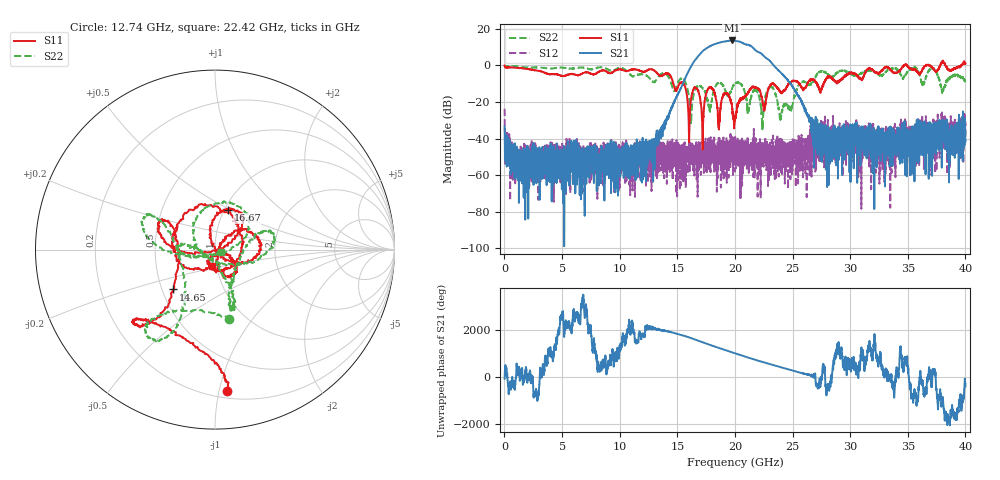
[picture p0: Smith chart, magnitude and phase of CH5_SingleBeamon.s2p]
!Keysight Technologies,N5245B,MY57181321,A.14.80.03
!Date: Thursday, March 28, 2024 19:43:59
!Correction: S11(C  2-Port  )
!S21(C  2-Port  )
!S12(C  2-Port  )
!S22(C  2-Port  )
!S2P File: Measurements: S11, S21, S12, S22:
# Hz S  RI  R 50
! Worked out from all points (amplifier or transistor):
!   4000 points, 10 MHz to 40 GHz, reference 50 ohm
!   highest |S21| = 13.7 dB at 19.73 GHz (marker M1)
!   |S21| within 3 dB of that: 17.88 GHz to 21.39 GHz (3.51 GHz wide, 17.9 % of centre)
!   unconditionally stable (mu >= 1): 15.4 MHz to 34.65 GHz; 34.96 GHz to 36.55 GHz; 38.27 GHz to 39.61 GHz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
!   at 6.67 GHz: K = 26125.73, MAG = -37.4 dB, |S12| = -65.4 dB
!   at 20.01 GHz: K = 76.01, MAG = 14.0 dB, |S12| = -58.1 dB
!   at 40 GHz: K = -267.43, MSG = -2.7 dB, |S12| = -30.6 dB
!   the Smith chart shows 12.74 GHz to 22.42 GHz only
!   S11 on the Smith chart (normalised r, x): 12.74 GHz: 0.25, -1.06; 14.65 GHz: 0.57, -0.28; 16.67 GHz: 1.04, +0.49; 22.42 GHz: 0.95, -0.17
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1e7  0.9943 -0.0372  0.00504 -0.0208  -0.055 0.0347  -0.9791 0.0426
6.68e9  0.2945 0.5044  -0.00285 -0.00276  -0.00171 -0.00146  0.8145 0.3385
1.274e10  0.0662 -0.7879  0.00294 -0.00392  -0.00284 0.000729  0.0805 -0.3877
1.334e10  -0.0625 -0.571  -0.00795 -0.0119  -0.000748 0.00354  -0.3036 -0.3661
1.465e10  -0.2313 -0.2218  -0.0057 0.0864  0.00161 -0.00291  -0.1835 -0.1164
1.611e10  0.0674 0.0272  -0.4226 -0.7262  0.00366 -0.00125  -0.0462 -0.0377
1.667e10  0.0734 0.2219  -1.217 1.015  -0.00259 0.00216  0.1898 0.1756
1.711e10  -0.0185 0.0458  1.125 2.017  -0.000644 -0.00199  -0.00339 0.2543
1.755e10  0.1736 -0.0702  2.863 -0.837  0.000278 0.00117  -0.119 0.0703
1.807e10  0.2062 0.0929  -1.03 -3.501  0.000312 -0.00505  0.1388 -0.0831
1.859e10  0.0193 0.00379  -4.067 0.9829  0.000737 -0.0101  0.3317 0.0573
1.914e10  0.0942 -0.1418  0.9517 4.452  -0.00117 -0.00257  0.208 0.062
1.973e10  0.076 -0.0301  4.538 -1.675  0.000994 -0.00389  0.0814 -0.2065
2.001e10  -0.000619 -0.0329  1.866 -4.324  0.0012 0.000336  0.0885 -0.3174
2.062e10  0.0595 -0.1036  -4.035 -1.188  -0.000324 -0.000391  0.0975 -0.2664
2.121e10  0.1154 0.1617  -0.5398 3.583  0.000394 0.00263  -0.0543 -0.0235
2.175e10  -0.2085 0.1426  2.551 0.7771  -0.00595 0.00101  -0.2069 0.00516
2.242e10  -0.0168 -0.0891  0.2964 -1.906  -0.00221 -0.00123  0.034 -0.0116
2.355e10  -0.1593 0.2265  -0.3883 0.7794  -0.00663 0.000959  0.00409 0.1549
2.667e10  0.1387 0.3834  0.0012 0.0287  0.0182 0.00104  0.0313 0.3326
3.334e10  0.4474 0.7281  -0.0192 -0.00607  -0.0131 -0.00691  0.7318 -0.1963
4e10  0.9322 0.6449  0.0116 -0.0111  -0.0221 0.0196  0.0368 -0.3286
